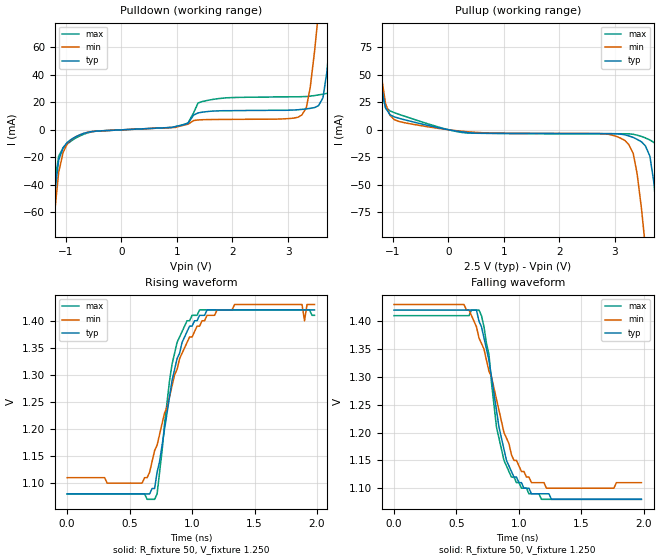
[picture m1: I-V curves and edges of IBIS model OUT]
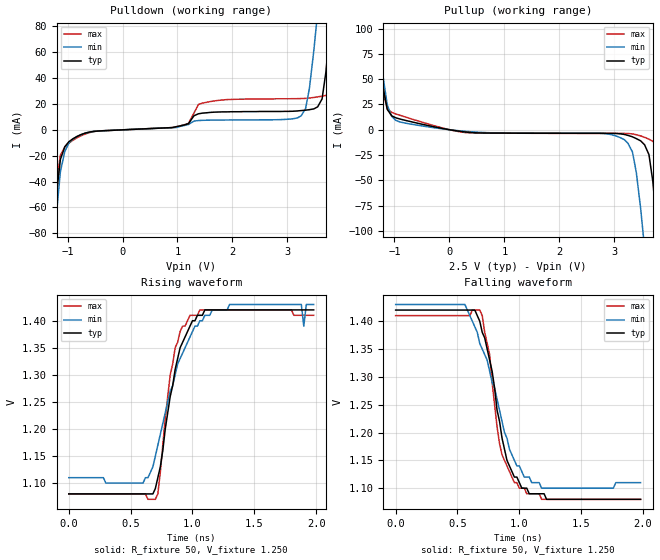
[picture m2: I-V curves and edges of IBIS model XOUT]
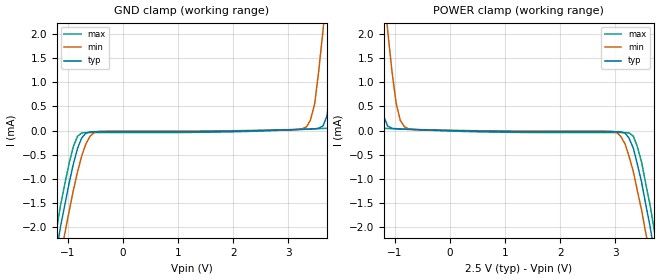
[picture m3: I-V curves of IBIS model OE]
| IBIS File sg7050van_25v.ibs
[IBIS Ver] 3.2
[File name] sg7050van_25v.ibs
[File Rev] 1
[Date] May 1 2013
[Source]
[Disclaimer]
Seiko Epson Corporation makes no warranty with respect to the information
contained herein.
[Copyright]
Copyright(C) 2013 Seiko Epson Corporation. All rights reserved.
| Component SG7050VAN 2.5V
[Component] sg7050van_25v
[Manufacturer] Seiko Epson Corporation
[Package]
R_pkg 0.224 NA NA
L_pkg 5.50n NA NA
C_pkg 1.45p NA NA
[Pin] signal_name model_name R_pin L_pin C_pin
1 OE OE
2 GND GND
3 GND GND
4 OUT OUT 0.224 5.50n 1.45p
5 XOUT XOUT 0.224 5.50n 1.45p
6 VCC POWER
[Diff Pin] inv_pin vdiff tdelay_typ
4 5 0 0
| Models and submodels in the file (3): OUT (Output), XOUT (Output), OE (Input)
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[Model] OUT
Model_type Output
Enable Active-High
Polarity Non-Inverting
Vref=1.250
Vmeas=1.250
Rref=50
Cref=0
C_comp 0.12p 0.12p 0.12p
[Temperature Range] 25 105 -40
[Voltage Range] 2.5 2.25 2.75
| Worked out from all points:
|   slope of the pulldown table from 0 to 0.375 V, typ, clamps not added: 511 ohm
|   slope of the pullup table from 0 to 0.375 V, typ, clamps not added: 139 ohm
|   falling waveform, R_fixture 50, V_fixture 1.250: 20-80 % time 166ps typ, 238ps min, 132ps max; typ from 1.42 V to 1.08 V
|   rising waveform, R_fixture 50, V_fixture 1.250: 20-80 % time 167ps typ, 248ps min, 111ps max; typ from 1.08 V to 1.42 V
[Pullup]
-2.5V     608mA      542mA      682mA
-1.38V    114mA      114mA      118mA
-1.13V    19.6mA     23.8mA     20.3mA
-900mV    10.6mA     7.69mA     14.2mA
3.18V     -4.61mA    -9.69mA    -3.65mA
3.33V     -7mA       -21.5mA    -4.12mA
3.55V     -14.7mA    -107mA     -7.47mA
3.63V     -23.9mA    -143mA     -9.27mA
3.8V      -99.2mA    -226mA     -15.2mA
3.88V     -139mA     -262mA     -21.2mA
4.1V      -261mA     -369mA     -125mA
5V        -746mA     -797mA     -669mA
[Pulldown]
-2.5V     -752mA     -684mA     -825mA
-1.3V     -98mA      -107mA     -93.3mA
-1.13V    -22.2mA    -31mA      -19.2mA
-825mV    -5.11mA    -5.19mA    -6.08mA
3.18V     14.5mA     9.05mA     23.9mA
3.33V     15.1mA     16mA       24.1mA
3.55V     17.5mA     85.8mA     25.3mA
3.63V     23.2mA     114mA      25.8mA
3.8V      85mA       180mA      27.5mA
3.95V     151mA      237mA      43.2mA
4.03V     183mA      265mA      76.8mA
5V        610mA      635mA      564mA
[Falling Waveform]
R_fixture=50
V_fixture=1.250
V_fixture_min=1.271
V_fixture_max=1.238
0s        1.42V      1.43V      1.41V
560ps     1.42V      1.43V      1.41V
660ps     1.42V      1.39V      1.42V
680ps     1.4V       1.37V      1.42V
760ps     1.33V      1.31V      1.34V
820ps     1.24V      1.26V      1.21V
880ps     1.17V      1.2V       1.15V
960ps     1.12V      1.15V      1.12V
1.1ns     1.09V      1.11V      1.09V
1.98ns    1.08V      1.11V      1.08V
[Rising Waveform]
R_fixture=50
V_fixture=1.250
V_fixture_min=1.271
V_fixture_max=1.238
0s        1.08V      1.11V      1.08V
600ps     1.08V      1.1V       1.08V
700ps     1.09V      1.16V      1.07V
720ps     1.12V      1.17V      1.08V
840ps     1.29V      1.28V      1.32V
1ns       1.39V      1.37V      1.41V
1.34ns    1.42V      1.43V      1.42V
1.88ns    1.42V      1.43V      1.42V
1.9ns     1.42V      1.4V       1.42V
1.98ns    1.42V      1.43V      1.41V
[Ramp]
R_load=50
dV/dt_r 2.043E-1/1.691E-10 1.915E-1/2.577E-10 2.027E-1/1.141E-10
dV/dt_f 2.042E-1/1.705E-10 1.920E-1/2.307E-10 2.021E-1/1.392E-10
|[End OUT
[Model] XOUT
Model_type Output
Enable Active-High
Polarity Inverting
Vref=1.250
Vmeas=1.250
Rref=50
Cref=0
C_comp 0.12p 0.12p 0.12p
[Temperature Range] 25 105 -40
[Voltage Range] 2.5 2.25 2.75
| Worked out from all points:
|   slope of the pulldown table from 0 to 0.375 V, typ, clamps not added: 511 ohm
|   slope of the pullup table from 0 to 0.375 V, typ, clamps not added: 139 ohm
|   falling waveform, R_fixture 50, V_fixture 1.250: 20-80 % time 166ps typ, 242ps min, 132ps max; typ from 1.42 V to 1.08 V
|   rising waveform, R_fixture 50, V_fixture 1.250: 20-80 % time 152ps typ, 248ps min, 106ps max; typ from 1.08 V to 1.42 V
[Pullup]
-2.5V     654mA      577mA      741mA
-1.38V    123mA      121mA      128mA
-1.13V    20.1mA     24.6mA     20.6mA
-900mV    10.6mA     7.71mA     14.3mA
3.18V     -4.61mA    -9.72mA    -3.65mA
3.33V     -7.01mA    -22mA      -4.12mA
3.55V     -14.8mA    -117mA     -7.5mA
3.63V     -24.6mA    -156mA     -9.3mA
3.8V      -109mA     -247mA     -15.3mA
3.88V     -154mA     -286mA     -21.6mA
4.1V      -288mA     -403mA     -140mA
5V        -826mA     -872mA     -750mA
[Pulldown]
-2.5V     -833mA     -748mA     -926mA
-1.3V     -108mA     -117mA     -104mA
-1.13V    -23mA      -32.5mA    -19.6mA
-825mV    -5.13mA    -5.2mA     -6.12mA
3.18V     14.5mA     9.08mA     24mA
3.33V     15.1mA     16.3mA     24.2mA
3.55V     17.7mA     91.3mA     25.4mA
3.63V     23.8mA     121mA      25.9mA
3.8V      91.4mA     192mA      27.7mA
3.95V     162mA      252mA      45.7mA
4.03V     197mA      282mA      83.5mA
5V        655mA      676mA      613mA
[Falling Waveform]
R_fixture=50
V_fixture=1.250
V_fixture_min=1.271
V_fixture_max=1.238
0s        1.42V      1.43V      1.41V
560ps     1.42V      1.43V      1.41V
680ps     1.4V       1.36V      1.42V
760ps     1.33V      1.31V      1.34V
820ps     1.24V      1.26V      1.21V
860ps     1.19V      1.22V      1.16V
900ps     1.15V      1.19V      1.14V
1.02ns    1.1V       1.13V      1.1V
1.18ns    1.09V      1.1V       1.08V
1.98ns    1.08V      1.11V      1.08V
[Rising Waveform]
R_fixture=50
V_fixture=1.250
V_fixture_min=1.271
V_fixture_max=1.238
0s        1.08V      1.11V      1.08V
600ps     1.08V      1.1V       1.08V
700ps     1.09V      1.15V      1.07V
860ps     1.31V      1.3V       1.35V
980ps     1.39V      1.37V      1.41V
1.3ns     1.42V      1.43V      1.42V
1.88ns    1.42V      1.43V      1.41V
1.9ns     1.42V      1.39V      1.41V
1.92ns    1.42V      1.43V      1.41V
1.98ns    1.42V      1.43V      1.41V
[Ramp]
R_load=50
dV/dt_r 2.043E-1/1.603E-10 1.916E-1/2.419E-10 2.026E-1/1.110E-10
dV/dt_f 2.042E-1/1.740E-10 1.921E-1/2.418E-10 2.021E-1/1.313E-10
|[End XOUT
[Model] OE
Model_type Input
Vinh=1.75
Vinl=0.75
C_comp 3p 3p 3p
[Temperature Range] 25 105 -40
[Voltage Range] 2.5 2.25 2.75
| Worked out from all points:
|   GND clamp passes 1 mA (typ) near -0.96 V on its own axis
|   POWER clamp passes 1 mA (typ) near -1.29 V on its own axis
[GND Clamp]
-2.5V     -11.7mA    -12.2mA    -11.3mA
-1.2V     -2.44mA    -3.04mA    -2mA
-1.05V    -1.5mA     -2.09mA    -1.07mA
-750mV    -154uA     -527uA     -50uA
-450mV    -23.9uA    -19.1uA    -41.7uA
3.33V     27.9uA     75.8uA     27.3uA
3.48V     35.3uA     560uA      34.9uA
3.63V     94uA       2.07mA     42.5uA
3.7V      295uA      2.97mA     46.5uA
3.88V     2.01mA     5.06mA     78.2uA
4.18V     5.9mA      8.64mA     2.74mA
5V        16.6mA     18.5mA     14.2mA
[POWER Clamp]
-2.5V     16.6mA     18.5mA     14.2mA
-1.68V    5.9mA      8.64mA     2.74mA
-1.38V    2.01mA     5.06mA     78.2uA
-1.2V     295uA      2.97mA     46.5uA
-1.13V    94uA       2.07mA     42.5uA
-975mV    35.3uA     560uA      34.9uA
-825mV    27.9uA     75.8uA     27.3uA
2.95V     -23.9uA    -19.1uA    -41.7uA
3.25V     -154uA     -527uA     -50uA
3.55V     -1.5mA     -2.09mA    -1.07mA
3.7V      -2.44mA    -3.04mA    -2mA
5V        -11.7mA    -12.2mA    -11.3mA
